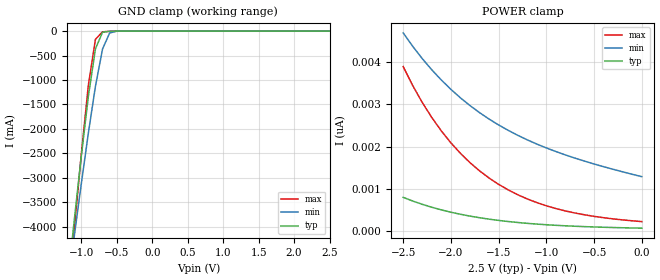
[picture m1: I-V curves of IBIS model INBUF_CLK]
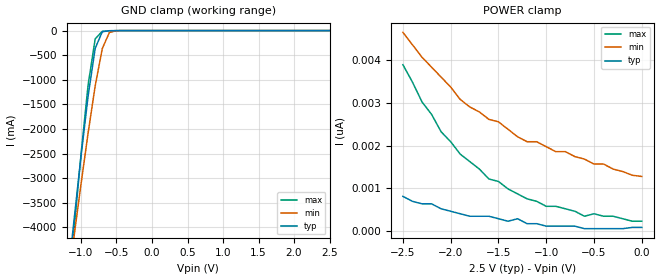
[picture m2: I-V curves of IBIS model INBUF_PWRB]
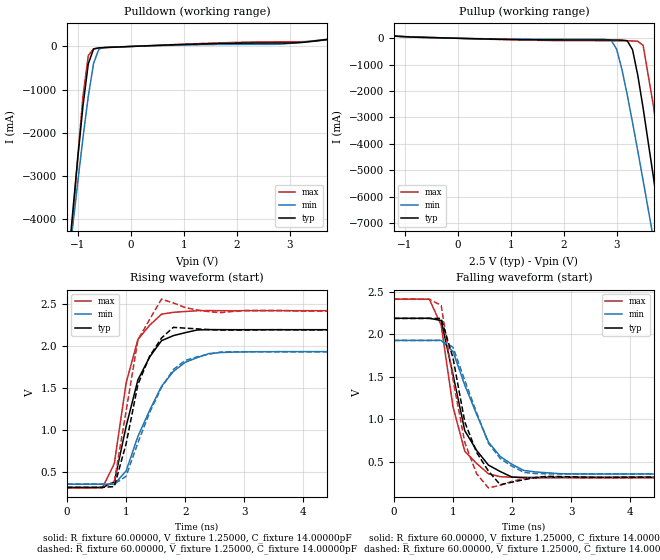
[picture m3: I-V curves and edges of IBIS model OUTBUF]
| IBIS file cspt857_tssop_2700.ibs created by s2ibis2 version 1.2
| North Carolina State University Electronics Research Laboratory  1995
[IBIS ver]   2.1
[File name]   cspt857_tssop_2700.ibs
[File Rev]   1.0
[Date]   Monday, August 25, 2003
[Source]   IDT
[Notes]   1. Temp typ=25C, min=0C, max=100C
   2. IDT's 2.0v C11.5 process
   3. Ramp rate based on 50 ohm load
READ THESE TERMS AND CONDITIONS CAREFULLY BEFORE USING THIS IBIS MODEL.  BY
USING THIS IBIS MODEL, YOU ARE ACCEPTING AND AGREEING TO THESE TERMS AND
CONDITIONS OF USE.
Integrated Device Technology, Inc. ("IDT") hereby grants the user of this
IBIS model ("User") a non-exclusive, nontransferable license to use this
IBIS model under the following terms: The User is granted this license only
to use the IBIS model for demonstration purposes only and is not granted
rights to sell, copy (except as needed to run the IBIS model), rent, lease
or sub-license (except for demonstration) the IBIS model in whole or in
part, or in modified form to anyone. The User may modify the IBIS model to
suit its specific applications, but  rights to derivative works and such
modifications shall belong to IDT.
THIS IBIS MODEL IS PROVIDED ON AN AS IS" BASIS AND IDT  MAKES ABSOLUTELY NO
WARRANTY WITH RESPECT TO THE INFORMATION CONTAINED HEREIN.  IDT DISCLAIMS
AND USER WAIVES ALL WARRANTIES, EXPRESS AND IMPLIED, INCLUDING WARRANTIES OF
MERCHANTABILITY AND FITNESS FOR A PARTICULAR PURPOSE.  THE ENTIRE RISK AS TO
QUALITY AND PERFORMANCE IS WITH THE USER  ACCORDINGLY, IN NO EVENT SHALL IDT
BE LIABLE FOR ANY DIRECT OR INDIRECT DAMAGES, WHETHER IN CONTRACT OR TORT,
INCLUDING ANY LOST PROFITS OR OTHER INCIDENTAL, CONSEQUENTIAL, EXEMPLARY, OR
PUNITIVE DAMAGES ARISING OUT OF THE USE OR APPLICATION OF THE  IBIS MODEL,
WHETHER OR NOT IDT HAD NOTICE OF SUCH DAMAGES.
IDT reserves the right to make changes without notice to any product herein
to improve
reliability, function, or design. IDT does not convey any license under
patent rights or any other intellectual property rights, including those of
third parties. IDT is not obligated
to provide maintenance or support for the licensed IBIS model.
This model is for the 2.5V Phase Locked Loop Differential 1:10 SDRAM Clock
Driver
[Copyright]
Copyright 2002, Integrated Device Technology, Inc. All rights reserved.
|   Component CPST857C
[Component]   CPST857C
[Manufacturer]   Integrated Device Technology Inc.
[Package]
|Following package parameters are for TSSOP 48 lead package
| variable   typ   min   max
R_pkg   0.10400   77.000000m   0.13000
L_pkg   3.20000nH   2.50000nH   4.40000nH
C_pkg   0.27000pF   0.17000pF   0.39000pF
[Pin]  signal_name   model_name   R_pin   L_pin   C_pin
1   GND   GND
2   _Y0_   OUTBUF
3   Y0   OUTBUF
4   VDDQ   POWER
5   Y1   OUTBUF
6   _Y1_   OUTBUF
7   GND   GND
8   GND   GND
9   _Y2_   OUTBUF
10   Y2   OUTBUF
11   VDDQ   POWER
12   VDDQ   POWER
13   CLK   INBUF_CLK
14   _CLK_   INBUF_CLK
15   VDDQ   POWER
16   AVDD   POWER
17   AGND   GND
18   GND   GND
19   _Y3_   OUTBUF
20   Y3   OUTBUF
21   VDDQ   POWER
22   Y4   OUTBUF
23   _Y4_   OUTBUF
24   GND   GND
25   GND   GND
26   _Y9_   OUTBUF
27   Y9   OUTBUF
28   VDDQ   POWER
29   Y8   OUTBUF
30   _Y8_   OUTBUF
31   GND   GND
32   FBOUT   OUTBUF
33   _FBOUT_   OUTBUF
34   VDDQ   POWER
35   _FBIN_   INBUF_FBIN
36   FBIN   INBUF_FBIN
37   _PWRDWN_   INBUF_PWRB
38   VDDQ   POWER
39   Y7   OUTBUF
40   _Y7_   OUTBUF
41   GND   GND
42   GND   GND
43   _Y6_   OUTBUF
44   Y6   OUTBUF
45   VDDQ   POWER
46   Y5   OUTBUF
47   _Y5_   OUTBUF
48   GND   GND
| in   in   dummy_model
| *oe  oe   dummy_model
[Diff Pin]  inv_pin  vdiff   tdelay_typ  tdelay_min  tdelay_max
13   14   1.00V   NA   |CLK<P:N> Clock Input pair
36   35   1.00V   NA   |FBIN<P:N> FBIN Input pair
3   2   0.000V   NA   |YX<P:N> Output pair
5   6   0.000V   NA   |YX<P:N> Output pair
10   9   0.000V   NA   |YX<P:N> Output pair
20   19   0.000V   NA   |YX<P:N> Output pair
22   23   0.000V   NA   |YX<P:N> Output pair
27   26   0.000V   NA   |YX<P:N> Output pair
29   30   0.000V   NA   |YX<P:N> Output pair
32   33   0.000V   NA   |YX<P:N> Output pair
39   40   0.000V   NA   |YX<P:N> Output pair
44   43   0.000V   NA   |YX<P:N> Output pair
46   47   0.000V   NA   |YX<P:N> Output pair
[Pin Mapping]  pulldown_ref   pullup_ref   gnd_clamp_ref  power_clamp_ref
1   GND   NC
2   GND   VDDQ
3   GND   VDDQ
4   NC   VDDQ
5   GND   VDDQ
6   GND   VDDQ
7   GND   NC
8   GND   NC
9   GND   VDDQ
10   GND   VDDQ
11   NC   VDDQ
12   NC   VDDQ
13   NC   NC   GND   VDDQ
14   NC   NC   GND   VDDQ
15   NC   VDDQ
16   NC   AVDD
17   AGND   NC
18   GND   NC
19   GND   VDDQ
20   GND   VDDQ
21   NC   VDDQ
22   GND   VDDQ
23   GND   VDDQ
24   GND   NC
25   GND   NC
26   GND   VDDQ
27   GND   VDDQ
28   NC   VDDQ
29   GND   VDDQ
30   GND   VDDQ
31   GND   NC
32   GND   VDDQ
33   GND   VDDQ
34   NC   VDDQ
35   NC   NC   GND   VDDQ
36   NC   NC   GND   VDDQ
37   NC   NC   GND   VDDQ
38   NC   VDDQ
39   GND   VDDQ
40   GND   VDDQ
41   GND   NC
42   GND   NC
43   GND   VDDQ
44   GND   VDDQ
45   NC   VDDQ
46   GND   VDDQ
47   GND   VDDQ
48   GND   NC
| Models and submodels in the file (4): INBUF_CLK (Input), INBUF_PWRB (Input), INBUF_FBIN (Input), OUTBUF (Output)
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|   Model INBUF_CLK
[Model]   INBUF_CLK
Model_type   Input
Polarity   Non-Inverting
Vinl =  0.80000V
Vinh =  2.00000V
C_comp   2.30000pF   2.30000pF   2.30000pF
[Temperature Range]   25.00000   100.00000   0.000
[Voltage Range]   2.50000V   2.30000V   2.70000V
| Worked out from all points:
|   GND clamp passes 1 mA (typ) near -0.52 V on its own axis
[GND_clamp]
| voltage   I(typ)   I(min)   I(max)
-2.5V     -23.89A    -20.36A    -27.98A
-1.2V     -5.248A    -5.316A    -5.713A
-1.1V     -3.884A    -4.209A    -4.089A
-1V       -2.564A    -3.127A    -2.526A
-900mV    -1.335A    -2.086A    -1.108A
-800mV    -361.3mA   -1.127A    -168.2mA
-700mV    -23.9mA    -365.3mA   -14.69mA
-600mV    -2.784mA   -39.09mA   -5.291mA
-500mV    -459.2uA   -2.159mA   -1.358mA
2.5V      71.27pA    1.402nA    195.1pA
[POWER_clamp]
| voltage   I(typ)   I(min)   I(max)
-2.5V     798.8pA    4.684nA    3.887nA
-2.4V     712pA      4.366nA    3.439nA
-2.3V     634.4pA    4.076nA    3.039nA
-2.2V     565pA      3.811nA    2.683nA
-2V       448.2pA    3.35nA     2.086nA
-1.8V     356pA      2.967nA    1.618nA
-1.7V     317.8pA    2.8nA      1.425nA
-1.5V     254.3pA    2.509nA    1.106nA
-1.2V     185.1pA    2.157nA    761.7pA
-900mV    138.7pA    1.881nA    534.7pA
-500mV    99.57pA    1.587nA    349.9pA
0V        71.27pA    1.288nA    226.3pA
|   Model INBUF_PWRB
[Model]   INBUF_PWRB
Model_type   Input
Polarity   Non-Inverting
Vinl =  0.80000V
Vinh =  2.00000V
C_comp   2.30000pF   2.30000pF   2.30000pF
[Temperature Range]   25.00000   100.00000   0.000
[Voltage Range]   2.50000V   2.30000V   2.70000V
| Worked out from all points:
|   GND clamp passes 1 mA (typ) near -0.52 V on its own axis
[GND_clamp]
| voltage   I(typ)   I(min)   I(max)
-2.5V     -23.88A    -20.35A    -27.98A
-1.2V     -5.247A    -5.316A    -5.712A
-1.1V     -3.884A    -4.209A    -4.088A
-1V       -2.564A    -3.127A    -2.526A
-900mV    -1.335A    -2.086A    -1.108A
-800mV    -361.3mA   -1.126A    -168.2mA
-700mV    -23.9mA    -365.3mA   -14.69mA
-600mV    -2.784mA   -39.09mA   -5.291mA
-500mV    -459.2uA   -2.159mA   -1.358mA
2.5V      87.31pA    1.397nA    232.8pA
[POWER_clamp]
| voltage   I(typ)   I(min)   I(max)
-2.5V     814.9pA    4.657nA    3.9nA
-2.3V     640.3pA    4.075nA    3.027nA
-2.1V     523.9pA    3.609nA    2.328nA
-1.9V     407.5pA    3.085nA    1.804nA
-1.6V     349.2pA    2.619nA    1.222nA
-1.5V     291pA      2.561nA    1.164nA
-1.3V     291pA      2.212nA    873.1pA
-1.2V     174.6pA    2.095nA    756.7pA
-1V       116.4pA    1.979nA    582.1pA
-600mV    58.21pA    1.688nA    349.2pA
-500mV    58.21pA    1.572nA    407.5pA
0V        87.31pA    1.281nA    232.8pA
|   Model OUTBUF
[Model]   OUTBUF
Model_type   Output
Polarity   Non-Inverting
Vmeas =  1.25000V
C_comp   4.80000pF   4.80000pF   4.80000pF
[Temperature Range]   25.00000   100.00000   0.000
[Voltage Range]   2.50000V   2.30000V   2.70000V
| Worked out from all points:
|   slope of the pulldown table from 0 to 0.375 V, typ, clamps not added: 20.3 ohm
|   slope of the pullup table from 0 to 0.375 V, typ, clamps not added: 20 ohm
|   rising waveform, R_fixture 60.00000, V_fixture 1.25000, C_fixture 14.00000pF: 20-80 % time 468ps typ, 633ps min, 341ps max; typ from 0.315 V to 2.19 V
|   rising waveform, R_fixture 60.00000, V_fixture 1.25000, C_fixture 14.00000pF: 20-80 % time 419ps typ, 591ps min, 299ps max; typ from 0.316 V to 2.19 V
|   falling waveform, R_fixture 60.00000, V_fixture 1.25000, C_fixture 14.00000pF: 20-80 % time 441ps typ, 581ps min, 335ps max; typ from 2.19 V to 0.315 V
|   falling waveform, R_fixture 60.00000, V_fixture 1.25000, C_fixture 14.00000pF: 20-80 % time 393ps typ, 533ps min, 318ps max; typ from 2.19 V to 0.316 V
[Pulldown]
| voltage   I(typ)   I(min)   I(max)
-2.5V     -24.02A    -20.48A    -28.11A
-1.3V     -6.698A    -6.489A    -7.44A
-1.1V     -3.936A    -4.25A     -4.147A
-1V       -2.612A    -3.164A    -2.58A
-900mV    -1.378A    -2.12A     -1.157A
-800mV    -400.3mA   -1.157A    -211.8mA
-700mV    -58.29mA   -391.9mA   -53.12mA
-600mV    -32.51mA   -62.11mA   -38.49mA
-500mV    -25.4mA    -21.54mA   -29.24mA
2.8V      81.34mA    52.63mA    108.7mA
3.2V      89.68mA    97.53mA    110.8mA
5V        376.9mA    361.1mA    377.2mA
[Pullup]
| voltage   I(typ)   I(min)   I(max)
-2.5V     286.8mA    273.7mA    294mA
-900mV    50.69mA    50.88mA    59.76mA
2.9V      -64.27mA   -81.77mA   -93.6mA
3V        -64.95mA   -412.9mA   -93.85mA
3.2V      -91.83mA   -2.145A    -95.98mA
3.3V      -434.2mA   -3.192A    -101.2mA
3.4V      -1.414A    -4.28A     -112.7mA
3.5V      -2.65A     -5.394A    -270mA
3.7V      -5.347A    -7.664A    -2.64A
3.9V      -8.156A    -9.969A    -5.841A
4.1V      -11.01A    -12.29A    -9.193A
5V        -24.08A    -22.88A    -24.72A
[Ramp]
| variable   typ   min   max
dV/dt_r   1.04760/0.15068n   0.82920/0.17415n   1.21080/0.13672n
dV/dt_f   1.05510/0.13771n   0.87414/0.16331n   1.18398/0.13634n
R_load = 50.00000
[Rising Waveform]
R_fixture = 60.00000
V_fixture = 1.25000
V_fixture_min = 1.15000
V_fixture_max = 1.35000
C_fixture = 14.00000pF
| time   V(typ)   V(min)   V(max)
0s        315.1mV    354mV      310.2mV
600ps     314.6mV    354mV      313.6mV
800ps     380.5mV    352.7mV    599.6mV
1ns       1.042V     511.7mV    1.557V
1.2ns     1.595V     922.9mV    2.076V
1.4ns     1.869V     1.235V     2.245V
1.6ns     2.061V     1.518V     2.376V
2ns       2.155V     1.803V     2.408V
2.6ns     2.192V     1.919V     2.417V
10ns      2.191V     1.93V      2.417V
[Rising Waveform]
R_fixture = 60.00000
V_fixture = 1.25000
V_fixture_min = 1.15000
V_fixture_max = 1.35000
C_fixture = 14.00000pF
R_dut = 0.10400
L_dut = 3.20000nH
C_dut = 0.27000pF
| time   V(typ)   V(min)   V(max)
0s        316.3mV    355mV      311.6mV
800ps     325.3mV    354.6mV    387mV
1ns       835mV      448.5mV    1.224V
1.2ns     1.54V      847.9mV    2.071V
1.4ns     1.877V     1.208V     2.317V
1.6ns     2.093V     1.506V     2.554V
1.8ns     2.219V     1.718V     2.509V
2ns       2.209V     1.825V     2.454V
2.6ns     2.188V     1.925V     2.393V
10ns      2.189V     1.929V     2.415V
[Falling Waveform]
R_fixture = 60.00000
V_fixture = 1.25000
V_fixture_min = 1.15000
V_fixture_max = 1.35000
C_fixture = 14.00000pF
| time   V(typ)   V(min)   V(max)
0s        2.191V     1.93V      2.417V
600ps     2.192V     1.93V      2.415V
800ps     2.164V     1.931V     2.108V
1ns       1.526V     1.799V     1.147V
1.2ns     864.3mV    1.401V     621.2mV
1.6ns     459.2mV    731.7mV    356.9mV
1.8ns     383.4mV    560.5mV    322.2mV
2.2ns     311.3mV    396mV      312.7mV
2.8ns     315.2mV    358.3mV    310.2mV
10ns      315.1mV    354mV      310.2mV
[Falling Waveform]
R_fixture = 60.00000
V_fixture = 1.25000
V_fixture_min = 1.15000
V_fixture_max = 1.35000
C_fixture = 14.00000pF
R_dut = 0.10400
L_dut = 3.20000nH
C_dut = 0.27000pF
| time   V(typ)   V(min)   V(max)
0s        2.189V     1.929V     2.415V
600ps     2.189V     1.929V     2.415V
800ps     2.189V     1.93V      2.343V
1ns       1.723V     1.85V      1.47V
1.2ns     967.7mV    1.458V     724.1mV
1.4ns     608.7mV    1.077V     357.2mV
1.6ns     388.6mV    717.6mV    190.6mV
1.8ns     227.6mV    537.8mV    220.7mV
2.4ns     312.3mV    358.4mV    311.5mV
10ns      316.3mV    355mV      311.6mV
